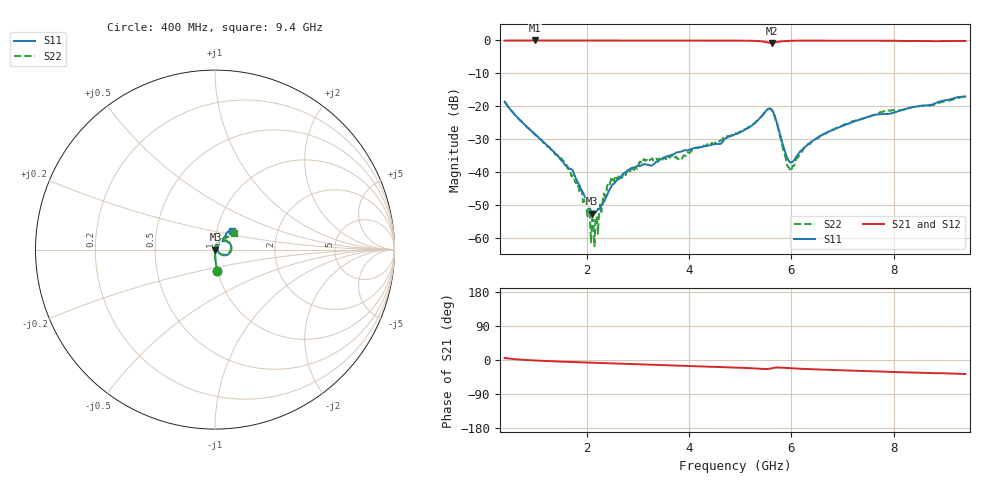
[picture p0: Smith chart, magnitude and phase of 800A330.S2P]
!  American Technical Ceramics  Date:  9/12/2007
!  One Norden Lane
!  Huntington Station,  NY.  11746-2102
!  Tel:  (631) 622-4700  Fax:  (631) 622-4748
!  Part Number  800A330  Mounting Orientation: Vertical
!  Description: Ultra Low ESR Microwave capacitors
!  Application: Coupling, Bypass, Tuning, DC Block
!  Filters, Matching
# GHZ S DB R 50
! Freq  |S11|  S11 Ph  |S21|  S21 Ph  |S12|  S12 Ph  |S22|  S22 Ph
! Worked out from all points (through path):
!   401 points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, 400 MHz to 9.4 GHz, reference 50 ohm
!   highest |S21| = -0.03 dB at 985 MHz (marker M1); lowest = -0.8 dB at 5.62 GHz (marker M2)
!   group delay of S21, straight-line fit = 11.7 ps
!   lowest |S11| = -52.6 dB at 2.11 GHz (marker M3), VSWR 1.00, Z = 50.2 - j0.0849 ohm
!   |S11| at or under -10 dB: start of sweep to end of sweep
!   |S22| runs from -62.5 to -17.0 dB; largest |S21 - S12| = 0.0038
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0.4  -18.60 -83.9  -0.08 5.4  -0.07 5.4  -18.56 -83.6
0.985  -28.37 -88.2  -0.03 -1.2  -0.02 -1.2  -28.48 -89.3
1.548  -37.07 -85.8  -0.03 -4.5  -0.02 -4.6  -36.86 -86.9
1.728  -39.45 -82.8  -0.04 -5.4  -0.03 -5.5  -40.96 -83.3
1.908  -45.56 -72.5  -0.03 -6.3  -0.03 -6.3  -45.76 -83.6
2.02  -49.74 -55.7  -0.04 -6.9  -0.03 -6.9  -53.41 -46.8
2.11  -52.62 -21.2  -0.04 -7.3  -0.03 -7.3  -54.09 -3.4
2.2  -51.73 8.6  -0.04 -7.7  -0.03 -7.7  -53.41 15.8
2.38  -47.61 53.5  -0.04 -8.5  -0.03 -8.6  -47.10 80.9
2.515  -43.66 60.5  -0.05 -9.2  -0.04 -9.2  -42.37 60.1
2.875  -38.87 63.9  -0.06 -10.7  -0.05 -10.8  -38.72 73.6
3.168  -37.72 74.0  -0.06 -12.0  -0.05 -12.1  -36.49 61.9
3.415  -36.50 83.9  -0.05 -13.0  -0.04 -13.1  -35.95 62.8
3.82  -33.84 77.9  -0.07 -14.8  -0.06 -14.9  -35.52 68.1
4.608  -31.41 69.8  -0.08 -18.4  -0.07 -18.5  -30.42 75.2
4.9  -28.55 63.8  -0.08 -19.7  -0.07 -19.8  -28.41 69.0
5.62  -21.08 -7.4  -0.82 -21.7  -0.82 -21.8  -21.23 -2.8
5.958  -36.73 -6.2  -0.15 -21.5  -0.14 -21.6  -38.62 1.0
6.408  -30.63 52.4  -0.08 -24.4  -0.08 -24.5  -30.57 62.5
7.218  -24.69 55.0  -0.10 -28.2  -0.10 -28.3  -24.56 58.3
7.915  -22.29 51.2  -0.11 -31.3  -0.12 -31.4  -21.32 48.0
9.4  -17.04 49.1  -0.19 -36.9  -0.20 -37.1  -16.99 40.2
